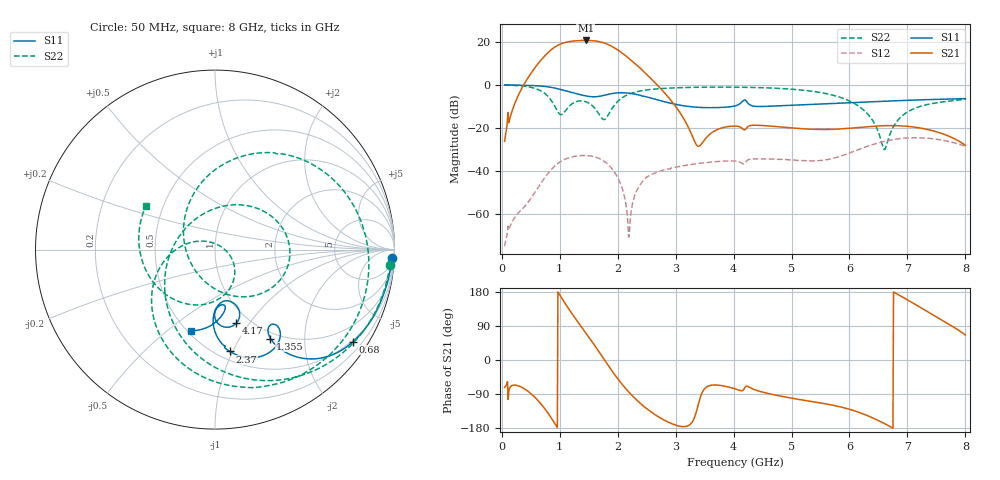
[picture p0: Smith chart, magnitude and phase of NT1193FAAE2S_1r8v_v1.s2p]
! Created Mon Jun 26 14:52:50 2023
# hz S ma R 50
! 2 Port Network Data from SP9.SP block
! freq  magS11  angS11  magS21  angS21  magS12  angS12  magS22  angS22
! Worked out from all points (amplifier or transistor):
!   856 points, 50 MHz to 8 GHz, reference 50 ohm
!   highest |S21| = 20.6 dB at 1.45 GHz (marker M1)
!   |S21| within 3 dB of that: 921.6 MHz to 1.916 GHz (994.6 MHz wide, 70.1 % of centre)
!   unconditionally stable (mu >= 1): start of sweep to end of sweep
!   at 1.285 GHz: K = 1.48, MAG = 22.7 dB, |S12| = -33.2 dB
!   at 3.73 GHz: K = 71.42, MAG = -14.1 dB, |S12| = -35.8 dB
!   at 8 GHz: K = 213.73, MAG = -26.1 dB, |S12| = -28.6 dB
!   lowest NFmin = 0.43 dB at 580 MHz
!   S11 on the Smith chart (normalised r, x): 50 MHz: 12, -40; 680 MHz: 0.46, -3.25; 1.355 GHz: 0.91, -1.37; 2.37 GHz: 0.58, -0.98; 4.17 GHz: 0.86, -0.87; 8 GHz: 0.52, -0.61
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5e7  0.9866 -2.6  0.04837 -72.6  0.0001746 99.3  0.9815 -5.0
4.7e8  0.9583 -22.6  1.562 -84.6  0.001957 125.3  0.8845 -47.4
6.8e8  0.925 -33.7  3.75 -116.3  0.005177 132.2  0.711 -81.1
8.6e8  0.8611 -43.9  6.575 -154.2  0.01076 116.1  0.4185 -129.0
1.04e9  0.7556 -52.5  9.085 162.3  0.01701 88.8  0.203 119.0
1.21e9  0.6548 -56.9  10.24 122.8  0.02084 62.2  0.3557 34.4
1.355e9  0.584 -58.0  10.6 91.7  0.02226 40.9  0.418 -3.3
1.375e9  0.5755 -58.0  10.62 87.5  0.02235 38.1  0.4179 -7.9
1.45e9  0.5472 -57.3  10.66 71.8  0.02238 27.2  0.3999 -25.2
1.585e9  0.5217 -53.9  10.47 42.7  0.0212 6.9  0.303 -60.2
1.695e9  0.5376 -51.2  9.919 18.1  0.01878 -10.6  0.1905 -105.0
1.8e9  0.5783 -51.3  8.974 -5.8  0.01524 -27.7  0.1649 177.4
1.94e9  0.6321 -56.7  7.233 -36.7  0.009456 -49.6  0.3273 112.1
2.16e9  0.6399 -70.2  4.448 -79.0  0.001098 -88.4  0.5725 68.7
2.37e9  0.5735 -81.6  2.544 -111.3  0.0043 91.0  0.7044 44.7
2.7e9  0.4382 -90.7  0.9322 -149.5  0.009399 79.0  0.8016 20.4
3.38e9  0.2973 -83.6  0.03728 -123.9  0.01457 58.4  0.8684 -11.3
4.03e9  0.3207 -70.3  0.1084 -76.2  0.01661 36.5  0.8724 -36.0
4.17e9  0.4274 -73.9  0.09068 -79.0  0.0143 37.4  0.868 -41.3
5.35e9  0.3478 -81.4  0.09168 -109.7  0.01689 -42.4  0.7031 -97.3
6.68e9  0.4153 -91.5  0.1114 -173.9  0.05052 149.0  0.06 -4.5
8e9  0.4729 -106.6  0.03885 65.9  0.03704 26.5  0.4553 147.7
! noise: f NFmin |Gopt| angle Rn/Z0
5e+07  2.562  0.9654  2.935  16.68
1e+09  0.4938  0.699  35.71  0.2685
1.525e+09  0.7076  0.6366  51.16  0.264
2.3e+09  1.353  0.5378  72.24  0.2944
3.25e+09  15.55  0.3104  86.51  11.02
4.2e+09  14.55  0.444  83.1  11.37
5.15e+09  16.64  0.3378  81.91  15.59
6.1e+09  18.96  0.3823  86.84  27.28
7.05e+09  18.61  0.4307  94.8  24.8
8e+09  26.19  0.4739  106.4  128.6
